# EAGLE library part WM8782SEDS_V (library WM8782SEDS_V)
Audio A/D Converter ICs STEREO ADC 20-pin Source: Datasheet
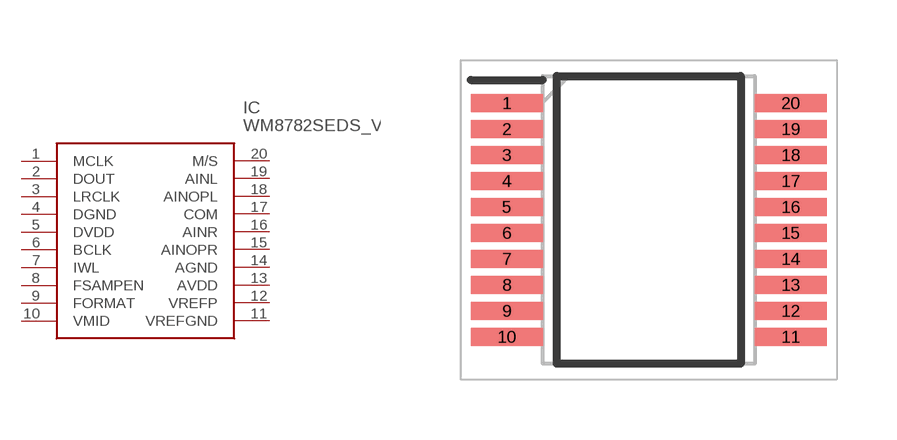
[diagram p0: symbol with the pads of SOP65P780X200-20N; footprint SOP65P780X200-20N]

Designator prefix IC

## WM8782SEDS_V (Description: Audio A/D Converter ICs STEREO ADC 20-pin; Height: 2mm; Manufacturer_Name: Cirrus Logic; Manufacturer_Part_Number: WM8782SEDS/V; Mouser_Part_Number: 238-WM8782SEDS/V; Mouser_Price-Stock: https://www.mouser.co.uk/ProductDetail/Cirrus-Logic/WM8782SEDS-V?qs=AjlVVxtvkmSRUSy8eTslnA%3D%3D)  [SOP65P780X200-20N]
1  MCLK
2  DOUT
3  LRCLK
4  DGND
5  DVDD
6  BCLK
7  IWL
8  FSAMPEN
9  FORMAT
10  VMID
11  VREFGND
12  VREFP
13  AVDD
14  AGND
15  AINOPR
16  AINR
17  COM
18  AINOPL
19  AINL
20  M/S

## Footprint SOP65P780X200-20N (pad centres in mm)
20pinssop
smd 1.8 x 0.45: 1 -3.55,2.925; 2 -3.55,2.275; 3 -3.55,1.625; 4 -3.55,0.975; 5 -3.55,0.325; 6 -3.55,-0.325; 7 -3.55,-0.975; 8 -3.55,-1.625; 9 -3.55,-2.275; 10 -3.55,-2.925; 11 3.55,-2.925; 12 3.55,-2.275; 13 3.55,-1.625; 14 3.55,-0.975; 15 3.55,-0.325; 16 3.55,0.325; 17 3.55,0.975; 18 3.55,1.625; 19 3.55,2.275; 20 3.55,2.925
